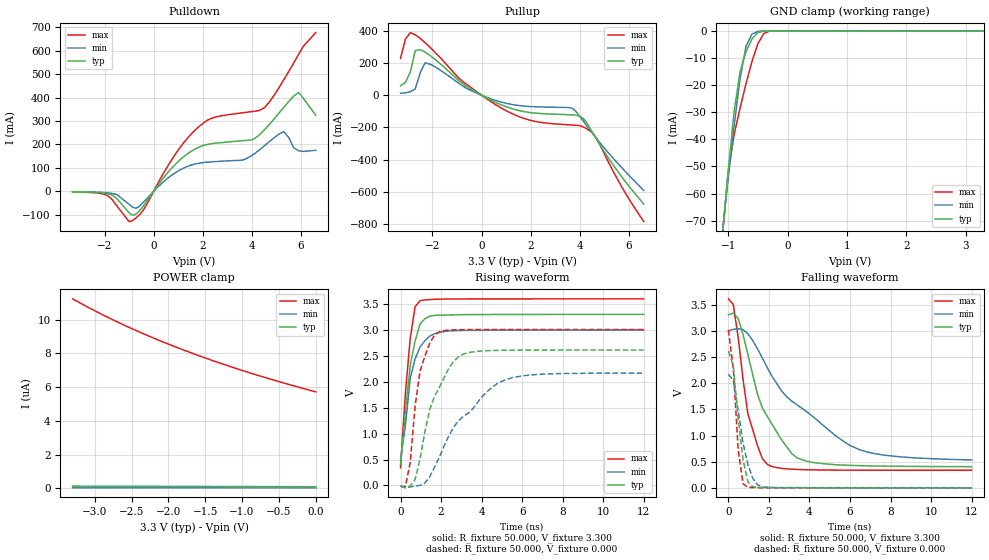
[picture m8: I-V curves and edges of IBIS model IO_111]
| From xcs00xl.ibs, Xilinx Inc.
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|   Model IO_111
[Model]   IO_111
Model_type   I/O
Polarity   Non-Inverting
Enable   Active-Low
Vinl =   0.800V
Vinh =   2.000V
Vmeas =   1.650V
Cref =  50.000pF
Rref =   1.000M
Vref =  0.000V
C_comp   5.300pF   3.500pF   6.800pF
[Temperature Range]   50.000   100.000   0.000
[Voltage Range]   3.300V   3.000V   3.600V
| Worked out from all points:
|   slope of the pulldown table from 0 to 0.495 V, typ, clamps not added: 7.07 ohm
|   slope of the pullup table from 0 to 0.495 V, typ, clamps not added: 12.6 ohm
|   GND clamp passes 1 mA (typ) near -0.52 V on its own axis
|   rising waveform, R_fixture 50.000, V_fixture 3.300: 20-80 % time 549ps typ, 596ps min, 413ps max; typ from 0.4 V to 3.3 V
|   rising waveform, R_fixture 50.000, V_fixture 0.000: 20-80 % time 1.19ns typ, 2.31ns min, 616ps max; typ from -0.013 V to 2.61 V
|   falling waveform, R_fixture 50.000, V_fixture 3.300: 20-80 % time 1.67ns typ, 3.56ns min, 842ps max; typ from 3.31 V to 0.405 V
|   falling waveform, R_fixture 50.000, V_fixture 0.000: 20-80 % time 432ps typ, 601ps min, 329ps max; typ from 2.62 V to 0 V
[Pulldown]
| voltage   I(typ)   I(min)   I(max)
-3.3V     -2.3mA     -1.8mA     -2.8mA
-1.9V     -9.7mA     -6.1mA     -16.3mA
-900mV    -100mA     -63.86mA   -127mA
-400mV    -59.92mA   -44.53mA   -76.62mA
700mV     94.99mA    66.07mA    129mA
1.6V      175mA      114mA      252mA
2.3V      202mA      125mA      309mA
3.6V      216mA      133mA      335mA
4.5V      261mA      193mA      356mA
5.3V      358mA      255mA      476mA
5.9V      422mA      173mA      584mA
6.6V      324mA      175mA      677mA
[Pullup]
| voltage   I(typ)   I(min)   I(max)
-3.3V     58.45mA    12.11mA    229mA
-3.1V     79.83mA    15.13mA    349mA
-2.9V     144mA      21.48mA    389mA
-2.7V     277mA      39.71mA    375mA
-2.5V     283mA      139mA      353mA
-2.1V     247mA      193mA      298mA
-800mV    74.73mA    60.76mA    89.48mA
900mV     -65.46mA   -46.11mA   -87.59mA
3.6V      -121mA     -77.38mA   -184mA
4V        -131mA     -132mA     -189mA
4.7V      -278mA     -272mA     -271mA
6.6V      -675mA     -591mA     -784mA
[GND_clamp]
| voltage   I(typ)   I(min)   I(max)
-3.3V     -539mA     -461mA     -635mA
-1.1V     -76.29mA   -74.81mA   -76.3mA
-1V       -51.66mA   -54.6mA    -52.25mA
-900mV    -29.77mA   -35.09mA   -38.23mA
-800mV    -15.1mA    -17.65mA   -28.49mA
-700mV    -7.645mA   -5.66mA    -19.53mA
-600mV    -2.968mA   -1.205mA   -11.34mA
-500mV    -649uA     -202uA     -4.68mA
-400mV    -83.34uA   -28.89uA   -976uA
-300mV    -8.303uA   -3.567uA   -95.2uA
3.3V      91.97nA    24.12nA    4.611uA
[POWER_clamp]
| voltage   I(typ)   I(min)   I(max)
-3.3V     126nA      27.82nA    11.23uA
-2.9V     121nA      27.69nA    10.3uA
-2.6V     117nA      27.28nA    9.671uA
-2.2V     113nA      27nA       8.903uA
-1.8V     109nA      25.98nA    8.207uA
-1.4V     104nA      25.34nA    7.571uA
-1V       101nA      24.85nA    6.988uA
-600mV    97.4nA     24.51nA    6.451uA
0V        91.96nA    23.79nA    5.718uA
[Ramp]
| variable   typ   min   max
dV/dt_r   1.567/1.192n   1.301/2.301n   1.805/0.602n
dV/dt_f   1.737/1.661n   1.479/3.552n   1.959/0.836n
R_load = 50.000
[Rising Waveform]
R_fixture = 50.000
V_fixture = 3.300
V_fixture_min = 3.000
V_fixture_max = 3.600
L_fixture = 0.000H
C_fixture = 0.000F
| time   V(typ)   V(min)   V(max)
0s        400mV      500mV      341mV
240ps     1.428V     1.148V     1.779V
480ps     2.319V     2.07V      2.843V
720ps     2.788V     2.442V     3.447V
960ps     3.108V     2.667V     3.563V
1.2ns     3.217V     2.791V     3.579V
1.44ns    3.265V     2.88V      3.585V
1.68ns    3.279V     2.928V     3.591V
2.4ns     3.289V     2.982V     3.596V
12ns      3.299V     2.999V     3.599V
[Rising Waveform]
R_fixture = 50.000
V_fixture = 0.000
V_fixture_min = 0.000
V_fixture_max = 0.000
L_fixture = 0.000H
C_fixture = 0.000F
| time   V(typ)   V(min)   V(max)
0s        -13.37mV   -9.16mV    -16.64mV
240ps     -43.22mV   -46.3mV    -22.03mV
480ps     -13.28mV   -28.53mV   446mV
720ps     115mV      -10.23mV   1.535V
960ps     505mV      -439uV     2.199V
1.44ns    1.464V     166mV      2.742V
1.92ns    1.895V     549mV      2.966V
2.88ns    2.487V     1.256V     3.004V
5.04ns    2.608V     2.016V     3.008V
12ns      2.612V     2.168V     3.009V
[Falling Waveform]
R_fixture = 50.000
V_fixture = 3.300
V_fixture_min = 3.000
V_fixture_max = 3.600
L_fixture = 0.000H
C_fixture = 0.000F
| time   V(typ)   V(min)   V(max)
0s        3.307V     3.004V     3.611V
240ps     3.338V     3.028V     3.5V
480ps     3.238V     3.039V     2.875V
960ps     2.547V     2.944V     1.416V
1.44ns    1.783V     2.653V     798mV
1.92ns    1.363V     2.293V     447mV
2.64ns    908mV      1.843V     371mV
3.36ns    581mV      1.592V     353mV
6.48ns    424mV      727mV      338mV
12ns      405mV      534mV      336mV
[Falling Waveform]
R_fixture = 50.000
V_fixture = 0.000
V_fixture_min = 0.000
V_fixture_max = 0.000
L_fixture = 0.000H
C_fixture = 0.000F
| time   V(typ)   V(min)   V(max)
0s        2.617V     2.172V     3.015V
240ps     2.33V      2.045V     2.28V
480ps     1.321V     1.483V     728mV
720ps     538mV      854mV      79.05mV
960ps     116mV      449mV      9.332mV
1.2ns     20.89mV    180mV      8.31mV
1.44ns    7.787mV    57.01mV    4.642mV
1.68ns    5.876mV    18.98mV    3.045mV
2.64ns    3.125mV    4.49mV     1.721mV
12ns      353uV      537uV      218uV
